| Texas Instruments Incorporated
| 6.4-GSPS Single-Channel or 3.2-GSPS Dual-Channel
| 12-Bit RF-Sampling Analog-to-Digital Converter (ADC)
| Marketing part#   ADC12DJ3200QML-SP
| Voltage Range   1.05V - 1.15V & 1.8V - 2.0V
| Package-type   CCGA [BGA]
| #pins/pkg drawing   196-pin NWE
| CCGA Ceramic Package with columns (ceramic column grid array)
[IBIS Ver]   4.1
[File name]   adc12dj3200qml-sp_ccga.ibs
[File Rev]   2.2
[Date]   12/15/2021
| Complete grounds-up generation of the IBIS model, therefore previous revision history deleted.
[Source]   Model built from spectre simulations at:
   Texas Instruments Incorporated.
   12500 TI Blvd
   Dallas, TX -75243
   Support: https://e2e.ti.com/support/data-converters/f/data-converters-forum
[Notes]
   Rev 2.0: 04/15/2021
   - all model data was revised
   - INPUT model now referring to VDD18
   - C_comp data was revised. Currently min and max values are sorted in numerical order
   (otherwise a warning is triggered by the syntax check).
   However, the max. C_comp value is derived for the IBIS min. case
   (high temp., low supply and weak process which leads to max. numerical C_comp value).
   Vice versa for min. C_comp.
   - prior NC models were replaced by TERMINATOR models which cover the clamping behaviour
   - RLC package data was revised
   - Vinl & Vinh in model SYNCB, DEVCLK and SYSREF refer to 1.1V supply
   Rev 2.1: 09/30/2021
   - corrected input pin list
   Rev 2.2: 12/15/2021
   - updates on PECL, LVDS models
   - update on OUTPUT model
[Disclaimer]  This model is designed as an aid for customers of Texas Instruments
 TI and its licensors and suppliers make no warranties, either expressed
 or implied, with respect to this  model, including the warranties of
 merchantability or fitness for a particular purpose.
 The model is provided solely on an "as is" basis. The entire risk as to
 its quality and performance is with the customer.
[Copyright] (C)Copyright 2021 Texas Instruments Incorporated.
   All rights reserved.
[Component]   ADC12DJ3200QML-SP_CCGA_PECL
[Manufacturer]  Texas Instruments Incorporated
[Package]   |196-pin ceramic BGA package
|   typ   min   max
R_pkg   1.49628   0.76337   2.44234
L_pkg   6.72n   5.21n   9.08n
C_pkg   2.35p   1.04p   3.28p
[Pin] signal_name  model_name   R_pin   L_pin   C_pin
A1   AGND   GND
A2   BG   BGCLAMP   1.32422   6.110E-09   2.750E-12
A3   AGND   GND
A4   INA+   ADCINCLAMP   1.57199   6.840E-09   1.927E-12
A5   INA-   ADCINCLAMP   1.57213   6.903E-09   1.923E-12
A6   AGND   GND
A7   NCOA0   INPUT   1.12265   5.645E-09   2.364E-12
A8   ORA0   OUTPUT   1.10867   6.175E-09   2.310E-12
A9   CALTRIG   INPUT   0.99458   6.173E-09   1.878E-12
A10   DA3+   DXCLAMP   1.47691   6.942E-09   2.009E-12
A11   DA3-   DXCLAMP   1.40641   6.866E-09   2.082E-12
A12   DA2+   DXCLAMP   1.86387   7.760E-09   2.544E-12
A13   DA2-   DXCLAMP   1.791   7.605E-09   2.601E-12
A14   DGND   GND
B1   AGND   GND
B2   SYNCSE\   INPUT   1.77118   6.823E-09   2.843E-12
B3   AGND   GND
B4   AGND   GND
B5   AGND   GND
B6   AGND   GND
B7   NCOA1   INPUT   0.97664   5.206E-09   2.214E-12
B8   ORA1   OUTPUT   0.95771   5.601E-09   2.109E-12
B9   CALSTAT   OUTPUT   0.76337   5.942E-09   1.043E-12
B10   DA7+   DXCLAMP   1.13418   5.749E-09   1.986E-12
B11   DA7-   DXCLAMP   1.11186   5.837E-09   2.017E-12
B12   DA6+   DXCLAMP   1.58589   6.943E-09   2.218E-12
B13   DA6-   DXCLAMP   1.57199   6.677E-09   2.351E-12
B14   DGND   GND
C1   TMSTP+   SYNCB_PECL   2.44234   9.023E-09   3.261E-12
C2   VA19   POWER
C3   VA19   POWER
C4   VA19   POWER
C5   VA19   POWER
C6   AGND   GND
C7   AGND   GND
C8   DGND   GND
C9   DGND   GND
C10   VD11   POWER
C11   VD11   POWER
C12   VD11   POWER
C13   DA5+   DXCLAMP   1.38389   6.253E-09   2.221E-12
C14   DA1+   DXCLAMP   1.79972   7.504E-09   2.394E-12
D1   TMSTP-   SYNCB_PECL   2.43825   9.079E-09   3.276E-12
D2   VA19   POWER
D3   VA11   POWER
D4   AGND   GND
D5   AGND   GND
D6   AGND   GND
D7   AGND   GND
D8   DGND   GND
D9   DGND   GND
D10   DGND   GND
D11   DGND   GND
D12   VD11   POWER
D13   DA5-   DXCLAMP   1.36348   6.396E-09   2.149E-12
D14   DA1-   DXCLAMP   1.73025   7.591E-09   2.344E-12
E1   VA19   POWER
E2   VA19   POWER
E3   VA11   POWER
E4   AGND   GND
E5   AGND   GND
E6   AGND   GND
E7   AGND   GND
E8   DGND   GND
E9   DGND   GND
E10   DGND   GND
E11   DGND   GND
E12   VD11   POWER
E13   DA4+   DXCLAMP   1.09954   5.713E-09   1.910E-12
E14   DA0+   DXCLAMP   1.40375   6.573E-09   1.872E-12
F1   AGND   GND
F2   VA11   POWER
F3   VA11   POWER
F4   AGND   GND
F5   AGND   GND
F6   AGND   GND
F7   AGND   GND
F8   DGND   GND
F9   DGND   GND
F10   DGND   GND
F11   DGND   GND
F12   VD11   POWER
F13   DA4-   DXCLAMP   1.08316   5.601E-09   2.051E-12
F14   DA0-   DXCLAMP   1.27044   6.404E-09   2.069E-12
G1   CLK+   DEVCLK_PECL   1.79259   7.041E-09   2.618E-12
G2   AGND   GND
G3   VA11   POWER
G4   AGND   GND
G5   AGND   GND
G6   AGND   GND
G7   AGND   GND
G8   DGND   GND
G9   DGND   GND
G10   DGND   GND
G11   DGND   GND
G12   VD11   POWER
G13   SCS\   INPUT   1.76744   6.746E-09   2.850E-12
G14   SCLK   INPUT   1.81476   7.013E-09   2.908E-12
H1   CLK-   DEVCLK_PECL   1.79279   7.036E-09   2.635E-12
H2   AGND   GND
H3   VA11   POWER
H4   AGND   GND
H5   AGND   GND
H6   AGND   GND
H7   AGND   GND
H8   DGND   GND
H9   DGND   GND
H10   DGND   GND
H11   DGND   GND
H12   VD11   POWER
H13   SDI   INPUT   1.77579   6.772E-09   2.848E-12
H14   SDO   OUTPUT   1.90177   7.194E-09   3.007E-12
J1   AGND   GND
J2   VA11   POWER
J3   VA11   POWER
J4   AGND   GND
J5   AGND   GND
J6   AGND   GND
J7   AGND   GND
J8   DGND   GND
J9   DGND   GND
J10   DGND   GND
J11   DGND   GND
J12   VD11   POWER
J13   DB4-   DXCLAMP   1.08427   5.602E-09   2.053E-12
J14   DB0-   DXCLAMP   1.27227   6.395E-09   2.057E-12
K1   VA19   POWER
K2   VA19   POWER
K3   VA11   POWER
K4   AGND   GND
K5   AGND   GND
K6   AGND   GND
K7   AGND   GND
K8   DGND   GND
K9   DGND   GND
K10   DGND   GND
K11   DGND   GND
K12   VD11   POWER
K13   DB4+   DXCLAMP   1.10236   5.719E-09   1.936E-12
K14   DB0+   DXCLAMP   1.40369   6.578E-09   1.869E-12
L1   SYSREF+   SYSREF_PECL   2.42168   8.841E-09   3.280E-12
L2   VA19   POWER
L3   VA11   POWER
L4   AGND   GND
L5   AGND   GND
L6   AGND   GND
L7   AGND   GND
L8   DGND   GND
L9   DGND   GND
L10   DGND   GND
L11   DGND   GND
L12   VD11   POWER
L13   DB5-   DXCLAMP   1.36362   6.401E-09   2.169E-12
L14   DB1-   DXCLAMP   1.73069   7.572E-09   2.357E-12
M1   SYSREF-   SYSREF_PECL   2.4243   8.601E-09   3.284E-12
M2   VA19   POWER
M3   VA19   POWER
M4   VA19   POWER
M5   VA19   POWER
M6   AGND   GND
M7   AGND   GND
M8   DGND   GND
M9   DGND   GND
M10   VD11   POWER
M11   VD11   POWER
M12   VD11   POWER
M13   DB5+   DXCLAMP   1.38478   6.246E-09   2.258E-12
M14   DB1+   DXCLAMP   1.80123   7.495E-09   2.413E-12
N1   AGND   GND
N2   TDIODE+   TDCLAMP   2.02949   7.228E-09   3.278E-12
N3   AGND   GND
N4   AGND   GND
N5   AGND   GND
N6   AGND   GND
N7   NCOB1   INPUT   1.01195   5.286E-09   2.392E-12
N8   ORB1   OUTPUT   0.89058   5.294E-09   2.191E-12
N9   DGND   GND
N10   DB7+   DXCLAMP   1.13523   5.752E-09   1.980E-12
N11   DB7-   DXCLAMP   1.1123   5.836E-09   2.016E-12
N12   DB6+   DXCLAMP   1.5869   6.938E-09   2.212E-12
N13   DB6-   DXCLAMP   1.56961   6.682E-09   2.334E-12
N14   DGND   GND
P1   AGND   GND
P2   TDIODE-   TDCLAMP   2.0299   7.272E-09   3.258E-12
P3   AGND   GND
P4   INB+   ADCINCLAMP   1.5719   6.786E-09   1.937E-12
P5   INB-   ADCINCLAMP   1.5723   6.780E-09   1.946E-12
P6   AGND   GND
P7   NCOB0   INPUT   1.1081   5.849E-09   2.490E-12
P8   ORB0   OUTPUT   1.00831   5.957E-09   2.331E-12
P9   PD   INPUT   0.94693   6.860E-09   1.639E-12
P10   DB3+   DXCLAMP   1.47544   6.941E-09   1.980E-12
P11   DB3-   DXCLAMP   1.40637   6.836E-09   2.083E-12
P12   DB2+   DXCLAMP   1.86281   7.759E-09   2.534E-12
P13   DB2-   DXCLAMP   1.79122   7.588E-09   2.601E-12
P14   DGND   GND
[Diff pin]  inv_pin  vdiff  tdelay_typ  tdelay_min  tdelay_max
A4   A5   0.0   0.0s   0.0s   0.0s   | INA
A10   A11   0.0   0.0s   0.0s   0.0s   | DA3
A12   A13   0.0   0.0s   0.0s   0.0s   | DA2
B10   B11   0.0   0.0s   0.0s   0.0s   | DA7
B12   B13   0.0   0.0s   0.0s   0.0s   | DA6
C1   D1   0.0   0.0s   0.0s   0.0s   | TMSTP
C13   D13   0.0   0.0s   0.0s   0.0s   | DA5
C14   D14   0.0   0.0s   0.0s   0.0s   | DA1
E13   F13   0.0   0.0s   0.0s   0.0s   | DA4
E14   F14   0.0   0.0s   0.0s   0.0s   | DA0
G1   H1   0.0   0.0s   0.0s   0.0s   | DEVCLK
K13   J13   0.0   0.0s   0.0s   0.0s   | DB4
K14   J14   0.0   0.0s   0.0s   0.0s   | DB0
L1   M1   0.0   0.0s   0.0s   0.0s   | SYSREF
M13   L13   0.0   0.0s   0.0s   0.0s   | DB5
M14   L14   0.0   0.0s   0.0s   0.0s   | DB1
N10   N11   0.0   0.0s   0.0s   0.0s   | DB7
N12   N13   0.0   0.0s   0.0s   0.0s   | DB6
P4   P5   0.0   0.0s   0.0s   0.0s   | INB
P10   P11   0.0   0.0s   0.0s   0.0s   | DB3
P12   P13   0.0   0.0s   0.0s   0.0s   | DB2
[Component]   ADC12DJ3200QML-SP_CCGA_LVDS
[Manufacturer]  Texas Instruments Incorporated
[Package]   |196-pin ceramic BGA package
|   typ   min   max
R_pkg   1.49628   0.76337   2.44234
L_pkg   6.72n   5.21n   9.08n
C_pkg   2.35p   1.04p   3.28p
[Pin] signal_name  model_name   R_pin   L_pin   C_pin
A1   AGND   GND
A2   BG   BGCLAMP   1.32422   6.110E-09   2.750E-12
A3   AGND   GND
A4   INA+   ADCINCLAMP   1.57199   6.840E-09   1.927E-12
A5   INA-   ADCINCLAMP   1.57213   6.903E-09   1.923E-12
A6   AGND   GND
A7   NCOA0   INPUT   1.12265   5.645E-09   2.364E-12
A8   ORA0   OUTPUT   1.10867   6.175E-09   2.310E-12
A9   CALTRIG   INPUT   0.99458   6.173E-09   1.878E-12
A10   DA3+   DXCLAMP   1.47691   6.942E-09   2.009E-12
A11   DA3-   DXCLAMP   1.40641   6.866E-09   2.082E-12
A12   DA2+   DXCLAMP   1.86387   7.760E-09   2.544E-12
A13   DA2-   DXCLAMP   1.791   7.605E-09   2.601E-12
A14   DGND   GND
B1   AGND   GND
B2   SYNCSE\   INPUT   1.77118   6.823E-09   2.843E-12
B3   AGND   GND
B4   AGND   GND
B5   AGND   GND
B6   AGND   GND
B7   NCOA1   INPUT   0.97664   5.206E-09   2.214E-12
B8   ORA1   OUTPUT   0.95771   5.601E-09   2.109E-12
B9   CALSTAT   OUTPUT   0.76337   5.942E-09   1.043E-12
B10   DA7+   DXCLAMP   1.13418   5.749E-09   1.986E-12
B11   DA7-   DXCLAMP   1.11186   5.837E-09   2.017E-12
B12   DA6+   DXCLAMP   1.58589   6.943E-09   2.218E-12
B13   DA6-   DXCLAMP   1.57199   6.677E-09   2.351E-12
B14   DGND   GND
C1   TMSTP+   SYNCB_LVDS   2.44234   9.023E-09   3.261E-12
C2   VA19   POWER
C3   VA19   POWER
C4   VA19   POWER
C5   VA19   POWER
C6   AGND   GND
C7   AGND   GND
C8   DGND   GND
C9   DGND   GND
C10   VD11   POWER
C11   VD11   POWER
C12   VD11   POWER
C13   DA5+   DXCLAMP   1.38389   6.253E-09   2.221E-12
C14   DA1+   DXCLAMP   1.79972   7.504E-09   2.394E-12
D1   TMSTP-   SYNCB_LVDS   2.43825   9.079E-09   3.276E-12
D2   VA19   POWER
D3   VA11   POWER
D4   AGND   GND
D5   AGND   GND
D6   AGND   GND
D7   AGND   GND
D8   DGND   GND
D9   DGND   GND
D10   DGND   GND
D11   DGND   GND
D12   VD11   POWER
D13   DA5-   DXCLAMP   1.36348   6.396E-09   2.149E-12
D14   DA1-   DXCLAMP   1.73025   7.591E-09   2.344E-12
E1   VA19   POWER
E2   VA19   POWER
E3   VA11   POWER
E4   AGND   GND
E5   AGND   GND
E6   AGND   GND
E7   AGND   GND
E8   DGND   GND
E9   DGND   GND
E10   DGND   GND
E11   DGND   GND
E12   VD11   POWER
E13   DA4+   DXCLAMP   1.09954   5.713E-09   1.910E-12
E14   DA0+   DXCLAMP   1.40375   6.573E-09   1.872E-12
F1   AGND   GND
F2   VA11   POWER
F3   VA11   POWER
F4   AGND   GND
F5   AGND   GND
F6   AGND   GND
F7   AGND   GND
F8   DGND   GND
F9   DGND   GND
F10   DGND   GND
F11   DGND   GND
F12   VD11   POWER
F13   DA4-   DXCLAMP   1.08316   5.601E-09   2.051E-12
F14   DA0-   DXCLAMP   1.27044   6.404E-09   2.069E-12
G1   CLK+   DEVCLK_LVDS   1.79259   7.041E-09   2.618E-12
G2   AGND   GND
G3   VA11   POWER
G4   AGND   GND
G5   AGND   GND
G6   AGND   GND
G7   AGND   GND
G8   DGND   GND
G9   DGND   GND
G10   DGND   GND
G11   DGND   GND
G12   VD11   POWER
G13   SCS\   INPUT   1.76744   6.746E-09   2.850E-12
G14   SCLK   INPUT   1.81476   7.013E-09   2.908E-12
H1   CLK-   DEVCLK_LVDS   1.79279   7.036E-09   2.635E-12
H2   AGND   GND
H3   VA11   POWER
H4   AGND   GND
H5   AGND   GND
H6   AGND   GND
H7   AGND   GND
H8   DGND   GND
H9   DGND   GND
H10   DGND   GND
H11   DGND   GND
H12   VD11   POWER
H13   SDI   INPUT   1.77579   6.772E-09   2.848E-12
H14   SDO   OUTPUT   1.90177   7.194E-09   3.007E-12
J1   AGND   GND
J2   VA11   POWER
J3   VA11   POWER
J4   AGND   GND
J5   AGND   GND
J6   AGND   GND
J7   AGND   GND
J8   DGND   GND
J9   DGND   GND
J10   DGND   GND
J11   DGND   GND
J12   VD11   POWER
J13   DB4-   DXCLAMP   1.08427   5.602E-09   2.053E-12
J14   DB0-   DXCLAMP   1.27227   6.395E-09   2.057E-12
K1   VA19   POWER
K2   VA19   POWER
K3   VA11   POWER
K4   AGND   GND
K5   AGND   GND
K6   AGND   GND
K7   AGND   GND
K8   DGND   GND
K9   DGND   GND
K10   DGND   GND
K11   DGND   GND
K12   VD11   POWER
K13   DB4+   DXCLAMP   1.10236   5.719E-09   1.936E-12
K14   DB0+   DXCLAMP   1.40369   6.578E-09   1.869E-12
L1   SYSREF+   SYSREF_LVDS   2.42168   8.841E-09   3.280E-12
L2   VA19   POWER
L3   VA11   POWER
L4   AGND   GND
L5   AGND   GND
L6   AGND   GND
L7   AGND   GND
L8   DGND   GND
L9   DGND   GND
L10   DGND   GND
L11   DGND   GND
L12   VD11   POWER
L13   DB5-   DXCLAMP   1.36362   6.401E-09   2.169E-12
L14   DB1-   DXCLAMP   1.73069   7.572E-09   2.357E-12
M1   SYSREF-   SYSREF_LVDS   2.4243   8.601E-09   3.284E-12
M2   VA19   POWER
M3   VA19   POWER
M4   VA19   POWER
M5   VA19   POWER
M6   AGND   GND
M7   AGND   GND
M8   DGND   GND
M9   DGND   GND
M10   VD11   POWER
M11   VD11   POWER
M12   VD11   POWER
M13   DB5+   DXCLAMP   1.38478   6.246E-09   2.258E-12
M14   DB1+   DXCLAMP   1.80123   7.495E-09   2.413E-12
N1   AGND   GND
N2   TDIODE+   TDCLAMP   2.02949   7.228E-09   3.278E-12
N3   AGND   GND
N4   AGND   GND
N5   AGND   GND
N6   AGND   GND
N7   NCOB1   INPUT   1.01195   5.286E-09   2.392E-12
N8   ORB1   OUTPUT   0.89058   5.294E-09   2.191E-12
N9   DGND   GND
N10   DB7+   DXCLAMP   1.13523   5.752E-09   1.980E-12
N11   DB7-   DXCLAMP   1.1123   5.836E-09   2.016E-12
N12   DB6+   DXCLAMP   1.5869   6.938E-09   2.212E-12
N13   DB6-   DXCLAMP   1.56961   6.682E-09   2.334E-12
N14   DGND   GND
P1   AGND   GND
P2   TDIODE-   TDCLAMP   2.0299   7.272E-09   3.258E-12
P3   AGND   GND
P4   INB+   ADCINCLAMP   1.5719   6.786E-09   1.937E-12
P5   INB-   ADCINCLAMP   1.5723   6.780E-09   1.946E-12
P6   AGND   GND
P7   NCOB0   INPUT   1.1081   5.849E-09   2.490E-12
P8   ORB0   OUTPUT   1.00831   5.957E-09   2.331E-12
P9   PD   INPUT   0.94693   6.860E-09   1.639E-12
P10   DB3+   DXCLAMP   1.47544   6.941E-09   1.980E-12
P11   DB3-   DXCLAMP   1.40637   6.836E-09   2.083E-12
P12   DB2+   DXCLAMP   1.86281   7.759E-09   2.534E-12
P13   DB2-   DXCLAMP   1.79122   7.588E-09   2.601E-12
P14   DGND   GND
[Diff pin]  inv_pin  vdiff  tdelay_typ  tdelay_min  tdelay_max
A4   A5   0.0   0.0s   0.0s   0.0s   | INA
A10   A11   0.0   0.0s   0.0s   0.0s   | DA3
A12   A13   0.0   0.0s   0.0s   0.0s   | DA2
B10   B11   0.0   0.0s   0.0s   0.0s   | DA7
B12   B13   0.0   0.0s   0.0s   0.0s   | DA6
C1   D1   0.0   0.0s   0.0s   0.0s   | TMSTP
C13   D13   0.0   0.0s   0.0s   0.0s   | DA5
C14   D14   0.0   0.0s   0.0s   0.0s   | DA1
E13   F13   0.0   0.0s   0.0s   0.0s   | DA4
E14   F14   0.0   0.0s   0.0s   0.0s   | DA0
G1   H1   0.0   0.0s   0.0s   0.0s   | DEVCLK
K13   J13   0.0   0.0s   0.0s   0.0s   | DB4
K14   J14   0.0   0.0s   0.0s   0.0s   | DB0
L1   M1   0.0   0.0s   0.0s   0.0s   | SYSREF
M13   L13   0.0   0.0s   0.0s   0.0s   | DB5
M14   L14   0.0   0.0s   0.0s   0.0s   | DB1
N10   N11   0.0   0.0s   0.0s   0.0s   | DB7
N12   N13   0.0   0.0s   0.0s   0.0s   | DB6
P4   P5   0.0   0.0s   0.0s   0.0s   | INB
P10   P11   0.0   0.0s   0.0s   0.0s   | DB3
P12   P13   0.0   0.0s   0.0s   0.0s   | DB2
[Series Pin Mapping]   pin_2   model_name   function_table_group
C1   D1   100_Ohm   | SYNCB/TMSTP with 100 Ohm termination
G1   H1   100_Ohm   | DEVCLK with 100 Ohm termination
L1   M1   100_Ohm   | SYSREF with 100 Ohm termination
[Model] 100_Ohm
Model_type Series
Polarity Non-Inverting
Enable Active-High
|   typ   min   max
C_comp   0   0   0
[Voltage Range]   1.10V   1.05V   1.15V
[Temperature Range]  25   125   -40
[R Series]   100   80   120
| Models and submodels in the file (13): SYNCB_LVDS (Input), SYNCB_PECL (Input), DEVCLK_LVDS (Input), DEVCLK_PECL (Input), SYSREF_LVDS (Input), SYSREF_PECL (Input), INPUT (Input), OUTPUT (3-state), DXCLAMP (Terminator), BGCLAMP (Terminator), TDCLAMP (Terminator), ADCINCLAMP (Terminator), 100_Ohm (Series)
